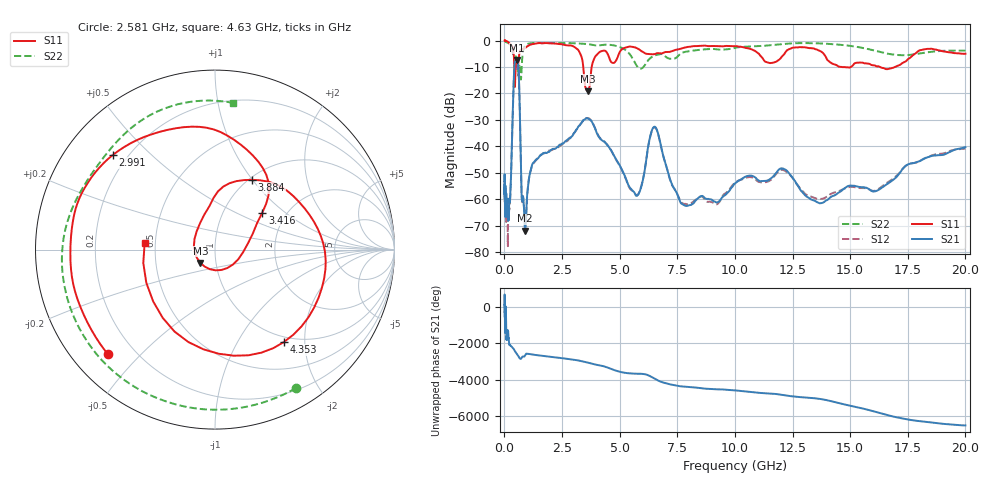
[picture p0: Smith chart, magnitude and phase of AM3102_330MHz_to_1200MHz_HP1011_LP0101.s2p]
! Date/Time: Tue, Sep 11, 2018 5:20 PM
! Network Analyzer: Agilent Technologies E8362B Rev: A.07.50.63
! Sweep from 0.010 to 20.000 GHz, 1601 Points, Sweep Type: LOG
! Power Supply: 4.949 V, 0.001 A
# Hz S DB R 50
!freq MagS11 AngS11 MagS21 AngS21 MagS12 AngS12 MagS22 AngS22
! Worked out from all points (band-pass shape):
!   1601 points, 10 MHz to 20 GHz, reference 50 ohm
!   highest |S21| = -7.32 dB at 553.8 MHz (marker M1); lowest = -71.9 dB at 903.4 MHz (marker M2)
!   |S21| within 3 dB of the highest: 432.1 MHz to 609.1 MHz (177 MHz wide, 34 % of centre)
!   lowest |S11| = -19.2 dB at 3.617 GHz (marker M3), VSWR 1.25, Z = 42 - j6.29 ohm
!   |S11| at or under -10 dB: 3.421 GHz to 3.788 GHz (367 MHz wide, 10.2 % of centre); 14.63 GHz to 15.03 GHz (397.4 MHz wide, 2.68 % of centre); 16.3 GHz to 16.95 GHz (654.7 MHz wide, 3.94 % of centre)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
!   |S22| runs from -14.8 to -0.2 dB; largest |S21 - S12| = 0.0063
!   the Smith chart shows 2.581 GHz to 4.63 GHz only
!   S11 on the Smith chart (normalised r, x): 2.581 GHz: 0.11, -0.40; 2.991 GHz: 0.15, +0.39; 3.416 GHz: 1.52, +0.70; 3.884 GHz: 1.03, +1.00; 4.353 GHz: 0.91, -1.60; 4.63 GHz: 0.44, +0.04
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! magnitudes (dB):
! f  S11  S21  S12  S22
! 10 MHz  0.0  -53.1  -55.1  -0.2
! 35.55 MHz  0.0  -66.4  -64.1  -0.3
! 126.4 MHz  -0.4  -65.7  -65.4  -0.8
! 147.8 MHz  -0.5  -63.9  -75.6  -0.9
! 260.2 MHz  -1.4  -57.2  -58.6  -1.6
! 447.2 MHz  -17.1  -8.7  -8.7  -6.4
! 553.8 MHz  -8.2  -7.3  -7.3  -8.7
! 635.6 MHz  -5.8  -15.6  -15.6  -10.2
! 754.2 MHz  -3.3  -59.4  -59.6  -9.6
! 903.4 MHz  -2.8  -71.9  -69.5  -1.9
! 1.59 GHz  -1.0  -43.2  -43.2  -0.9
! 2.581 GHz  -1.6  -38.7  -38.8  -1.0
! 2.991 GHz  -2.2  -35.4  -35.4  -1.0
! 3.416 GHz  -9.5  -30.2  -30.5  -1.2
! 3.617 GHz  -19.2  -29.5  -29.3  -1.4
! 3.884 GHz  -7.1  -32.2  -32.2  -1.8
! 4.353 GHz  -3.8  -38.4  -38.3  -1.6
! 4.63 GHz  -8.1  -41.5  -41.6  -1.7
! 5.652 GHz  -2.6  -57.7  -57.7  -8.2
! 6.487 GHz  -5.2  -32.7  -32.9  -5.8
! 7.92 GHz  -2.5  -62.6  -62.0  -4.2
! 20 GHz  -5.0  -40.3  -40.9  -3.8
